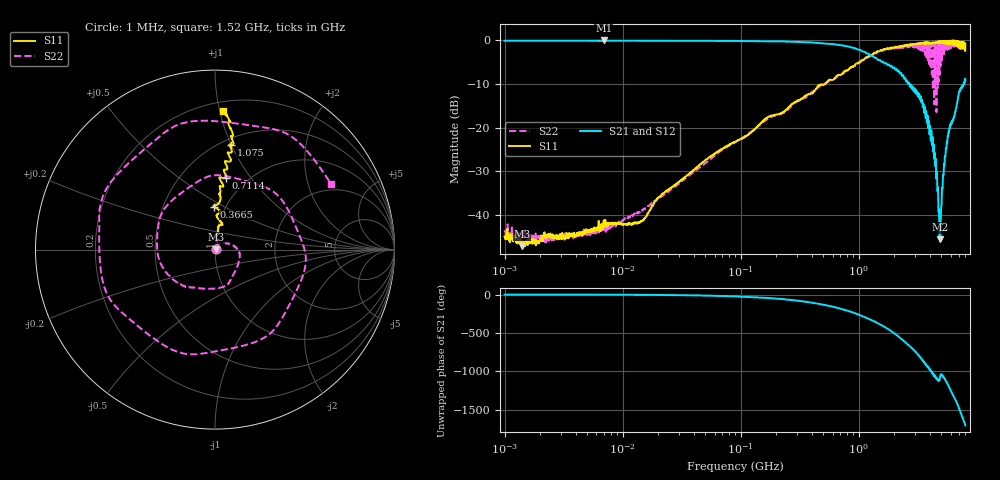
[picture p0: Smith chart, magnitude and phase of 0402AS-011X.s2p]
!s-Parameter Generated by FASTRON Sdn. Bhd.
!FASTRON P/N : 0402AS-011X
!Keysight Technologies: E5071C_MY46733604_B.14.02
!Date: Mon Dec 01 10:30:27 2025
!Version  :Rev00  Mon Dec 01 10:30:27 2025
!Data & Calibration Information:
!Freq  S11:SOLT2(ON)  S21:SOLT2(ON)  S12:SOLT2(ON)  S22:SOLT2(ON)
!PortZ  Port1:50+j0  Port2:50+j0
!When reading reference impedance value at option line is always used.
! Remarks : This data is being provided solely for informational purposes.
# Hz S dB R 50
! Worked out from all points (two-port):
!   1601 points, 1 MHz to 8 GHz, reference 50 ohm
!   highest |S21| = 0.00 dB at 6.912 MHz (marker M1); lowest = -45.5 dB at 4.856 GHz (marker M2)
!   |S21| within 3 dB of the highest: start of sweep to 1.177 GHz
!   lowest |S11| = -47.1 dB at 1.405 MHz (marker M3), VSWR 1.01, Z = 50.4 + j0.133 ohm
!   |S11| at or under -10 dB: start of sweep to 513.8 MHz
!   |S22| runs from -46.2 to -0.2 dB; largest |S21 - S12| = 0.017
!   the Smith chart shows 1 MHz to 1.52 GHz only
!   S11 on the Smith chart (normalised r, x): 1 MHz: 1.01, +0.00; 366.5 MHz: 0.88, +0.45; 711.4 MHz: 0.80, +0.77; 1.075 GHz: 0.56, +1.00; 1.52 GHz: 0.27, +1.03
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1000000  -44.90 16.9  -0.07 -0.3  -0.04 -0.3  -43.90 14.0
1404635  -47.10 17.4  -0.06 -0.4  -0.05 -0.4  -44.60 -1.9
4479405  -44.00 33.5  -0.06 -1.2  -0.05 -1.3  -44.50 34.8
6911657  -41.20 25.7  -0.00 -1.9  -0.03 -1.8  -41.50 31.3
2.00676e7  -36.00 56.4  -0.06 -5.5  -0.06 -5.4  -36.20 64.1
8.994653e7  -23.20 85.7  -0.12 -24.1  -0.11 -24.1  -23.30 31.1
3.664607e8  -12.40 91.4  -0.41 -96.8  -0.41 -96.8  -12.80 -110.0
4.006501e8  -12.10 89.1  -0.47 -106.0  -0.46 -106.0  -11.90 -125.0
7.113666e8  -7.84 81.6  -1.09 173.0  -1.09 173.0  -7.65 83.8
1.075264e9  -4.57 81.1  -2.48 78.7  -2.48 78.6  -4.40 -105.0
1.256741e9  -3.29 82.8  -3.46 33.0  -3.46 33.0  -3.34 161.0
1.519696e9  -2.26 86.5  -4.58 -30.1  -4.59 -30.2  -2.58 29.7
1.7949e9  -1.87 91.1  -5.50 -94.6  -5.51 -94.7  -2.03 -103.0
2.114474e9  -1.40 97.2  -6.81 -173.0  -6.80 -174.0  -1.68 93.4
2.486897e9  -1.14 102.0  -8.76 96.1  -8.74 96.0  -1.68 -93.1
2.853703e9  -1.02 109.0  -10.60 15.9  -10.60 15.7  -1.13 100.0
3.203473e9  -0.70 117.0  -13.00 -67.6  -12.90 -68.0  -0.76 -80.4
3.568312e9  -0.43 129.0  -16.10 -164.0  -16.00 -164.0  -2.33 70.8
3.933151e9  -0.70 132.0  -18.40 115.0  -18.30 115.0  -3.10 -73.6
4.856488e9  -0.19 151.0  -45.50 -4.9  -45.80 -3.5  -7.83 -143.0
5.304358e9  -0.72 173.0  -28.70 -12.9  -28.70 -12.9  -0.60 1.6
8e9  -0.69 -103.0  -9.09 97.9  -9.10 97.6  -2.15 133.0
